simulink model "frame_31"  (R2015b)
settings: Solver=FixedStepAuto  StartTime=0.0  StopTime=20  RelTol=1e-3
undefined symbols (not defined in the file or in its folder): fir1
libraries: dspsigops x4, simulink x1, dspstat3 x1

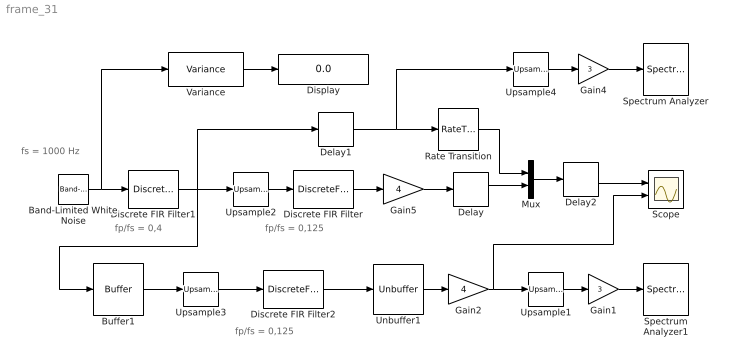
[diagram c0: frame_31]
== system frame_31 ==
  note: fp/fs = 0,125
  note: fp/fs = 0,4
  note: fs = 1000 Hz
  note: fp/fs = 0,125
  Band-Limited White Noise : simulink/Sources/Band-Limited White Noise  Cov=1/1000  Ts=1/1000  seed=[23341]
  Buffer1 : Buffer  N=2048  TreatMby1Signals=One channel  OutputFrames=off
  Delay : Delay  DelayLength=4*2048
  Delay1 : Delay  DelayLength=2048 +8
  Delay2 : Delay  DelayLength=5*2048-4
  Discrete FIR Filter : DiscreteFir  Coefficients=fir1(64, 0.25);
  Discrete FIR Filter1 : DiscreteFir  Coefficients=fir1(128, 0.8);
  Discrete FIR Filter2 : DiscreteFir  Coefficients=fir1(64, 0.25);  InputProcessing=Columns as channels (frame based)
  Display : Display
  Gain1 : Gain  Gain=3
  Gain2 : Gain  Gain=4
  Gain4 : Gain  Gain=3
  Gain5 : Gain  Gain=4
  Mux : Mux  Inputs=2
  Rate Transition : RateTransition
  Scope : Scope  NumInputPorts=2
  Spectrum Analyzer : SpectrumAnalyzer
  Spectrum Analyzer1 : SpectrumAnalyzer
  Unbuffer1 : Unbuffer  SampleBasedProcessing=Same as frame based
  Upsample1 : dspsigops/Upsample  N=3  phase=0  RateOptions=Allow multirate processing  ic=0  mode=Unused parameter value
  Upsample2 : dspsigops/Upsample  N=4  phase=0  RateOptions=Allow multirate processing  ic=0  mode=Unused parameter value
  Upsample3 : dspsigops/Upsample  N=4  phase=0  InputProcessing=Columns as channels (frame based)  RateOptions=Allow multirate processing  ic=0  mode=Unused parameter value
  Upsample4 : dspsigops/Upsample  N=3  phase=0  RateOptions=Allow multirate processing  ic=0  mode=Unused parameter value
  Variance : dspstat3/Variance  run=on  reset_popup=None  directionMode=Each column  dimension=1  roiEnable=off  roiType=Rectangles  roiPortion=Entire ROI  roiOutput=Individual statistics for each ROI  roiFlag=off  roundingMode=Floor  overflowMode=off
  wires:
  Band-Limited White Noise/1 -> Variance/1, Discrete FIR Filter1/1
  Variance/1 -> Display/1
  Buffer1/1 -> Upsample3/1
  Discrete FIR Filter2/1 -> Unbuffer1/1
  Unbuffer1/1 -> Gain2/1
  Discrete FIR Filter/1 -> Gain5/1
  Gain1/1 -> Spectrum Analyzer1/1
  Discrete FIR Filter1/1 -> Delay1/1, Upsample2/1, Buffer1/1
  Upsample2/1 -> Discrete FIR Filter/1
  Upsample3/1 -> Discrete FIR Filter2/1
  Gain2/1 -> Scope/2, Upsample1/1
  Upsample4/1 -> Gain4/1
  Upsample1/1 -> Gain1/1
  Gain5/1 -> Delay/1
  Delay/1 -> Mux/2
  Rate Transition/1 -> Mux/1
  Mux/1 -> Delay2/1
  Delay2/1 -> Scope/1
  Delay1/1 -> Rate Transition/1, Upsample4/1
  Gain4/1 -> Spectrum Analyzer/1
